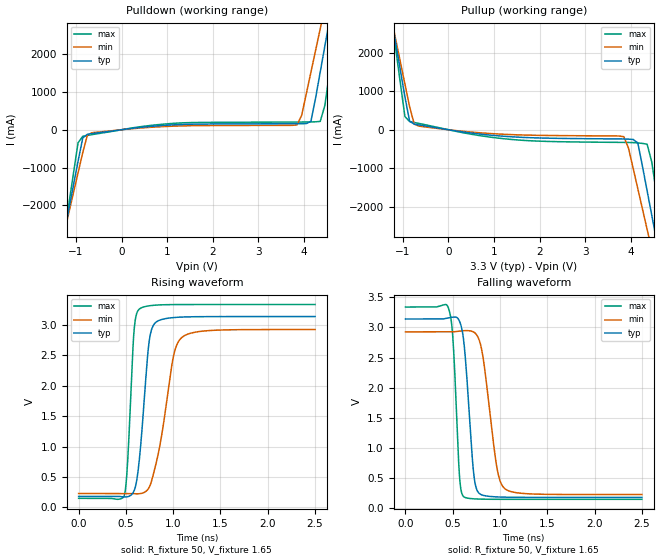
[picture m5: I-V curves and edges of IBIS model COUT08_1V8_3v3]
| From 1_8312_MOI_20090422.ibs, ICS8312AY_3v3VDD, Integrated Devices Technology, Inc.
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[Model] COUT08_1V8_3v3
Model_type   Output
Polarity   Non-Inverting
|   typ   min   max
C_comp   2pF   1.5pF   2.5pF
Vmeas = 1.65V
Rref = 50
Vref = 1.65V
|   typ   min   max
[Voltage range]   3.3V   3.135V   3.465V
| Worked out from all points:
|   slope of the pulldown table from 0 to 0.495 V, typ, clamps not added: 6.88 ohm
|   slope of the pullup table from 0 to 0.495 V, typ, clamps not added: 5.83 ohm
|   rising waveform, R_fixture 50, V_fixture 1.65: 20-80 % time 91.3ps typ, 165ps min, 57.6ps max; typ from 0.181 V to 3.14 V
|   falling waveform, R_fixture 50, V_fixture 1.65: 20-80 % time 79.4ps typ, 126ps min, 55.5ps max; typ from 3.14 V to 0.181 V
[pulldown]
|Voltage   I (typ)   I (min)   I (max)
-3.3V     -15.53A    -13.39A    -19.08A
-1.259V   -2.756A    -2.739A    -2.801A
-952.6mV  -833mA     -1.14A     -345.2mA
-850.5mV  -218.6mA   -607.6mA   -174.7mA
-646.4mV  -102mA     -79.42mA   -129.6mA
3.844V    159mA      127.2mA    203.8mA
4.151V    222.7mA    1.522A     206.6mA
4.355V    1.528A     2.671A     221.2mA
4.559V    2.913A     3.823A     1.532A
4.661V    3.607A     4.4A       2.419A
4.763V    4.301A     4.977A     3.307A
6.6V      17.06A     15.56A     19.6A
[pullup]
|Voltage   I (typ)   I (min)   I (max)
-3.3V     16.98A     14.61A     20.9A
-1.259V   2.959A     2.935A     3.016A
-952.6mV  850.4mA    1.182A     340.5mA
-850.5mV  221.4mA    597.4mA    213mA
-646.4mV  125.3mA    93.65mA    163.6mA
3.844V    -239.7mA   -179.7mA   -328.3mA
4.151V    -340.8mA   -1.527A    -342.5mA
4.355V    -1.582A    -2.581A    -373.9mA
4.457V    -2.217A    -3.11A     -836mA
4.661V    -3.487A    -4.167A    -2.459A
4.763V    -4.123A    -4.696A    -3.271A
6.6V      -15.57A    -14.23A    -17.87A
[Ramp]
|   typ   min   max
dV/dt_r   2.376/0.141n   2.163/0.251n   2.565/0.088n
dV/dt_f   2.393/0.121n   2.176/0.190n   2.586/0.086n
[Rising Waveform]
R_fixture = 50
V_fixture = 1.65
V_fixture_max = 1.73
V_fixture_min = 1.57
C_fixture = 0.0p
| Time   typ   min   max
0s        180.7mV    228.1mV    148.5mV
481.9ps   170.7mV    228.6mV    188.6mV
517.1ps   174.4mV    228.6mV    715mV
584.8ps   266.6mV    224.4mV    2.879V
642.6ps   790.3mV    224.5mV    3.264V
740.4ps   2.664V     313.6mV    3.317V
818.3ps   3.048V     717.1mV    3.329V
1.001ns   3.124V     2.476V     3.338V
1.094ns   3.133V     2.8V       3.339V
2.5ns     3.141V     2.927V     3.339V
[Falling Waveform]
R_fixture = 50
V_fixture = 1.65
V_fixture_max = 1.73
V_fixture_min = 1.57
C_fixture = 0.0p
| Time   typ   min   max
0s        3.141V     2.927V     3.339V
459.3ps   3.161V     2.926V     3.299V
504.5ps   3.172V     2.927V     2.744V
572.3ps   3.1V       2.939V     508.3mV
617.5ps   2.752V     2.946V     190.8mV
717.9ps   627.2mV    2.927V     157.1mV
780.6ps   245.4mV    2.786V     152.3mV
963.8ps   188.5mV    700.6mV    148.9mV
1.044ns   184.3mV    334.5mV    148.6mV
2.5ns     180.7mV    228.1mV    148.5mV
